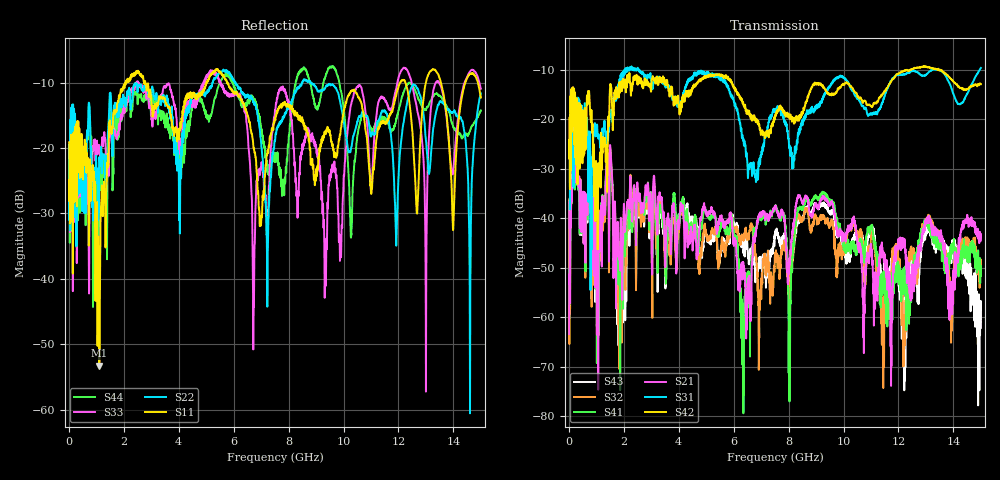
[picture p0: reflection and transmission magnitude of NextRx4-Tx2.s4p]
! FILE: N:\QM 2007\Prüfprotokolle\Highspeed\Konfektionierte Ltg\L45593-D106\D30\8216\0002\Next  Platine 1\NextRx4-Tx2.s4p
# MHz S DB R 50.00
! FREQ  S11  S12  S13  S14
!  S21  S22  S23  S24
!  S31  S32  S33  S34
!  S41  S42  S43  S44
!  DB  ANG  DB  ANG  DB  ANG  DB  ANG
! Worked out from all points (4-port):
!   2999 points, 10 MHz to 15 GHz, reference 50 ohm
!   strongest paths, dB at 10 MHz, 3.755 GHz, 7.505 GHz, 11.26 GHz, 15 GHz:
!     S42: -25.8, -13.5, -19.7, -16.3, -12.9
!     S31: -24.5, -15.5, -18.6, -18.4, -9.6
!     S21: -63.4, -38.8, -37.5, -51.9, -43.7
!     S41: -53.5, -39.5, -37.7, -48.5, -51.1
!     S32: -39.8, -39.7, -48.3, -53.6, -50.4
!     S43: -42.1, -39.7, -43.6, -49.3, -62.1
!   lowest |S11| = -53.3 dB at 1.11 GHz (marker M1), VSWR 1.00, Z = 50.1 + j0.205 ohm
!   |S11| at or under -10 dB: start of sweep to 2.07 GHz; 2.783 GHz to 5.009 GHz (2.227 GHz wide, 57.2 % of centre); 5.781 GHz to 12.07 GHz (6.285 GHz wide, 70.4 % of centre)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
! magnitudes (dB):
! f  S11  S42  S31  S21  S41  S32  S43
! 10 MHz  -19.1  -25.8  -24.5  -63.4  -53.5  -39.8  -42.1
! 175 MHz  -19.6  -20.9  -20.9  -29.0  -29.7  -28.8  -29.9
! 1.11 GHz  -53.3  -30.9  -23.8  -45.9  -44.7  -46.7  -45.3
! 2.48 GHz  -8.2  -12.3  -10.1  -34.5  -35.9  -35.8  -36.9
! 6.735 GHz  -20.0  -19.6  -29.8  -43.7  -42.5  -44.8  -46.0
! 7.725 GHz  -13.5  -17.8  -19.2  -38.9  -40.0  -47.7  -44.5
! 15 GHz  -12.3  -12.9  -9.6  -43.7  -51.1  -50.4  -62.1
